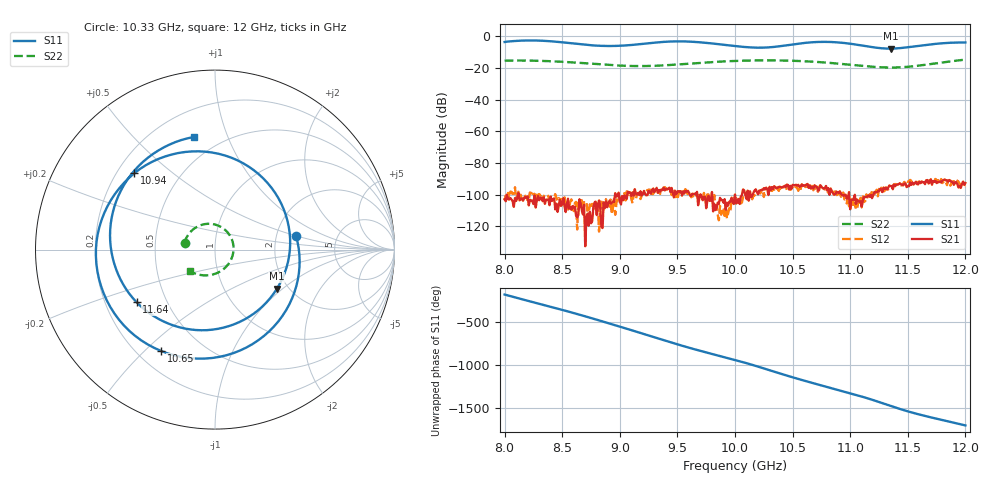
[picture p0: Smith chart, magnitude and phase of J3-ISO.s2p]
!Keysight Technologies,N5234A,MY52241180,A.10.60.03
!Date: Tuesday, May 30, 2023 15:18:51
!Correction: S11(Full 2 Port(1,2))
!S21(Full 2 Port(1,2))
!S12(Full 2 Port(1,2))
!S22(Full 2 Port(1,2))
!S2P File: Measurements: S11, S21, S12, S22:
# Hz S  dB  R 50
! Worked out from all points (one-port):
!   401 points, 8 GHz to 12 GHz, reference 50 ohm
!   lowest |S11| = -7.8 dB at 11.35 GHz (marker M1), VSWR 2.38, Z = 87.5 - j45.7 ohm
!   |S11| at or under -10 dB: nowhere
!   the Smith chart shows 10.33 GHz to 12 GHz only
!   S11 on the Smith chart (normalised r, x): 10.33 GHz: 2.59, +0.48; 10.65 GHz: 0.29, -0.56; 10.94 GHz: 0.27, +0.37; 11.64 GHz: 0.34, -0.27; 12 GHz: 0.36, +0.77
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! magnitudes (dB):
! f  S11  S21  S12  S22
! 8 GHz  -3.6  -103.0  -103.6  -15.4
! 8.15 GHz  -2.7  -102.4  -103.0  -15.3
! 8.29 GHz  -2.7  -101.0  -100.1  -15.5
! 8.67 GHz  -5.1  -109.9  -103.6  -16.9
! 8.96 GHz  -6.1  -99.2  -112.8  -18.3
! 9.15 GHz  -5.2  -100.1  -99.5  -18.8
! 9.34 GHz  -3.8  -97.1  -98.6  -18.5
! 9.61 GHz  -3.4  -100.5  -100.2  -17.2
! 10 GHz  -6.1  -100.0  -104.7  -15.6
! 10.18 GHz  -7.2  -96.7  -99.7  -15.2
! 10.33 GHz  -6.8  -96.7  -96.9  -15.2
! 10.65 GHz  -3.9  -94.1  -95.7  -15.9
! 10.67 GHz  -3.8  -95.4  -94.5  -16.0
! 10.81 GHz  -3.5  -95.9  -99.3  -16.7
! 10.94 GHz  -4.2  -100.7  -98.8  -17.6
! 11.23 GHz  -7.2  -98.7  -97.0  -19.4
! 11.34 GHz  -7.8  -94.2  -95.7  -19.7
! 11.35 GHz  -7.8  -94.6  -95.4  -19.7
! 11.48 GHz  -7.1  -93.0  -93.9  -19.4
! 11.64 GHz  -5.6  -92.2  -91.2  -18.1
! 11.83 GHz  -4.3  -91.1  -91.9  -16.2
! 12 GHz  -3.9  -92.7  -94.7  -14.7
